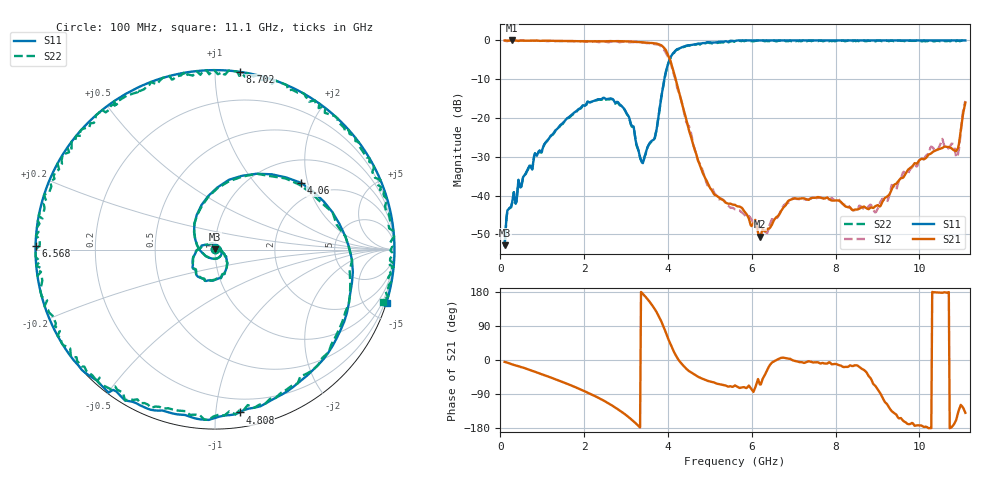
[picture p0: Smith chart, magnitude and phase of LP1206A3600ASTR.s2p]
!	AVX	THIN	FILM	OPERATION
!	LP1206	High	Performance	Low	Pass	Filters
!	P/N	LP1206A3600ASTR	14	September	2017
!Instrument:	"HEWLETT PACKARD,8720ES,US39172150,7.62 "
#	MHz	S	dB	R	50
!	Frq	S11(dB)	S11(deg)	S21(dB)	S21(deg)	S12(dB)	S12(deg)	S22(dB)	S22(deg)
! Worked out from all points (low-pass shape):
!   501 points, 100 MHz to 11.1 GHz, reference 50 ohm
!   highest |S21| = 0.00 dB at 276 MHz (marker M1); lowest = -50.6 dB at 6.194 GHz (marker M2)
!   |S21| within 3 dB of the highest: start of sweep to 3.971 GHz
!   lowest |S11| = -52.9 dB at 100 MHz (marker M3), VSWR 1.00, Z = 50.2 + j0.13 ohm
!   |S11| at or under -10 dB: start of sweep to 3.914 GHz
!   |S22| runs from -53.1 to 0.0 dB; largest |S21 - S12| = 0.063
!   S11 on the Smith chart (normalised r, x): 100 MHz: 1.00, +0.00; 4.06 GHz: 1.54, +1.82; 4.808 GHz: 0.10, -1.16; 6.568 GHz: -0.00, +0.01; 8.702 GHz: -0.00, +1.15; 11.1 GHz: -0.00, -6.63
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100  -52.86 34.7  0.00 -4.9  0.00 -3.7  -53.06 34.5
276  -42.04 18.2  0.00 -11.5  -0.02 -10.5  -42.04 18.1
848  -29.42 -10.8  -0.04 -32.2  -0.08 -32.4  -29.52 -10.9
1948  -16.98 -67.2  -0.21 -79.4  -0.20 -79.5  -17.08 -67.2
2828  -16.21 -143.5  -0.18 -131.9  -0.41 -132.2  -16.41 -143.6
3246  -26.74 140.6  -0.36 -168.6  -0.41 -168.2  -26.94 140.5
3400  -31.65 41.7  -0.48 174.5  -0.56 174.5  -31.75 41.5
3598  -26.05 -68.6  -0.65 148.2  -0.68 148.0  -26.15 -68.8
3774  -19.65 165.3  -0.95 116.8  -1.04 116.3  -19.65 165.3
3906  -10.42 97.1  -1.91 84.7  -2.36 83.7  -10.52 96.9
4060  -4.34 37.8  -5.31 42.0  -5.39 42.1  -4.54 37.6
4302  -1.90 -21.9  -14.95 -6.8  -14.87 -2.0  -1.90 -21.9
4808  -0.75 -81.4  -33.53 -48.8  -32.97 -50.6  -0.85 -81.4
5600  -0.15 -132.2  -42.41 -67.1  -43.57 -68.9  -0.15 -132.4
6194  0.00 -164.7  -50.59 -64.5  -48.10 -45.6  0.00 -164.8
6568  0.00 178.8  -45.82 -1.4  -46.08 -4.1  -0.20 178.7
7448  0.00 138.9  -40.60 -5.8  -40.77 -4.7  0.00 138.8
8702  0.00 82.0  -43.01 -28.5  -43.69 -33.9  -0.20 82.0
9274  0.00 57.7  -39.89 -124.6  -40.39 -116.2  -0.20 57.5
10286  0.00 16.5  -29.10 -179.8  -27.36 -175.8  0.00 16.4
10902  0.00 -10.2  -28.15 -148.9  -29.77 -157.3  0.00 -10.2
11100  0.00 -17.1  -16.05 -139.4  -15.60 -151.3  -0.20 -17.2
